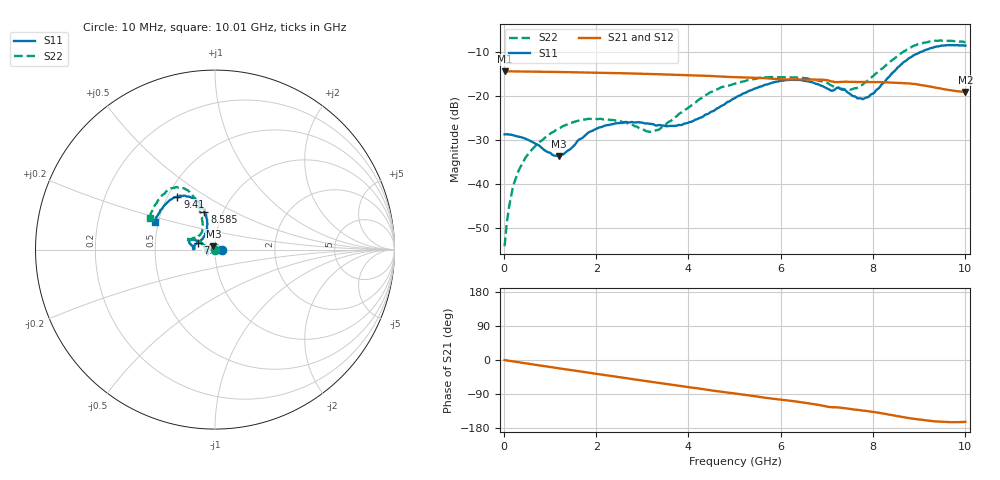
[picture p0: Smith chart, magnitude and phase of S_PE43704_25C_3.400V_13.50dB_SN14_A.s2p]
! Device ID: PE43704
! Dir: z:\PE43704\PE43704_Char_1_20130516\PE43704\AMB\3p400V\13p50dB
! Serial: 14
! Insertion: A
! Impedance: 50 ohm
! Temp: Amb
! VDD: 3.400V
! Attenuation Step: 13.50dB
! IDD: 1.139268e-01mA
#  Hz  S  RI  R  50
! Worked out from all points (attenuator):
!   401 points, 10 MHz to 10.01 GHz, reference 50 ohm
!   highest |S21| = -14.46 dB at 10 MHz (marker M1); lowest = -19.1 dB at 10.01 GHz (marker M2)
!   lowest |S11| = -33.7 dB at 1.185 GHz (marker M3), VSWR 1.04, Z = 49.1 + j1.83 ohm
!   |S11| at or under -10 dB: start of sweep to 9.069 GHz
!   |S22| runs from -54.1 to -7.5 dB; largest |S21 - S12| = 0.0015
!   S11 on the Smith chart (normalised r, x): 10 MHz: 1.08, +0.00; 7.51 GHz: 0.82, +0.06; 8.585 GHz: 0.82, +0.36; 9.41 GHz: 0.56, +0.38; 10.01 GHz: 0.48, +0.17
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1e7  0.0365 0.000299  0.1893 -0.000662  0.1894 -0.000703  0.00193 0.000393
1.6e8  0.0356 0.0061  0.1885 -0.0103  0.1886 -0.0102  0.00174 0.00743
2.35e8  0.0339 0.00914  0.188 -0.0148  0.188 -0.0147  0.000542 0.0109
3.6e8  0.0312 0.0134  0.1871 -0.0224  0.187 -0.0226  -0.00195 0.0157
6.85e8  0.0184 0.0216  0.1827 -0.0414  0.1826 -0.0413  -0.0126 0.0241
1.185e9  -0.00905 0.0186  0.1725 -0.0691  0.1725 -0.069  -0.0365 0.0214
1.685e9  -0.0329 0.00198  0.1579 -0.0942  0.1579 -0.0941  -0.0533 0.00525
2.435e9  -0.0435 -0.0221  0.1294 -0.1256  0.1294 -0.1256  -0.0507 -0.0114
3.135e9  -0.0411 -0.0256  0.0973 -0.1472  0.0973 -0.1471  -0.0392 -0.000722
3.36e9  -0.0415 -0.0212  0.0862 -0.1523  0.0865 -0.1522  -0.0407 0.00666
4.035e9  -0.0504 0.00203  0.0522 -0.1619  0.0525 -0.162  -0.0683 0.032
4.46e9  -0.0609 0.0193  0.0306 -0.1647  0.0309 -0.1649  -0.0946 0.0533
5.01e9  -0.0852 0.0402  0.00425 -0.1623  0.00464 -0.1623  -0.1257 0.0545
5.96e9  -0.1353 0.0553  -0.0373 -0.1496  -0.0366 -0.1497  -0.1534 0.0517
6.685e9  -0.1386 0.0311  -0.0663 -0.1373  -0.0663 -0.1373  -0.1445 0.052
7.51e9  -0.0974 0.0378  -0.0908 -0.1113  -0.0906 -0.1116  -0.0815 0.0846
7.86e9  -0.0629 0.0719  -0.1002 -0.1017  -0.1001 -0.1021  -0.069 0.1263
8.36e9  -0.044 0.1592  -0.1145 -0.0826  -0.1143 -0.0831  -0.0846 0.2215
8.585e9  -0.0594 0.2091  -0.1193 -0.0717  -0.1186 -0.0719  -0.1066 0.2722
8.935e9  -0.1048 0.275  -0.1235 -0.0552  -0.1229 -0.0539  -0.1639 0.3359
9.41e9  -0.2097 0.294  -0.1167 -0.0371  -0.1166 -0.0365  -0.2562 0.3316
1.001e10  -0.3353 0.1561  -0.1058 -0.0323  -0.1069 -0.0322  -0.3644 0.1769
